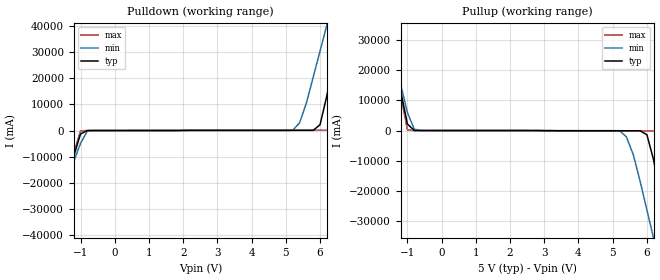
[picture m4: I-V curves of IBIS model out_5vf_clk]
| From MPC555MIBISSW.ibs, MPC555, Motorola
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| OUTPUT_5vf_clk(Full Strength, 90pf load)
[Model]   out_5vf_clk
Model_type   Output
Polarity   Non-Inverting
|   typ   min   max
C_comp   5.1000e-13   4.5360e-13   5.8450e-13
| CAP models
| typical : model= typ
| maximum : model= wcs
| minimum : model= bcs
[Voltage range]   5.0v   4.5v   5.5v
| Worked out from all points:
|   slope of the pulldown table from 0 to 0.75 V, typ, clamps not added: 187 ohm
|   slope of the pullup table from 0 to 0.75 V, typ, clamps not added: 744 ohm
|  typical: model = typ,  temp = 25,  vdd = 3.3, vddh = 5.0
|  maximum: model = bcs,  temp = -40, vdd = 3.6, vddh = 5.5
|  minimum: model = wcs,  temp = 150, vdd = 3.0, vddh = 4.5
[Pulldown]
|  Voltage   I(typ)   I(min)   I(max)
-5V       -319.1A    -223.2A    -410.6A
-1.8V     -50.29A    -40.81A    -60.01A
-1.6V     -36.77A    -31.17A    -42.83A
-1V       -1.324A    -4.896A    -109.6mA
5.2V      64.08mA    77.3mA     107mA
5.6V      64.46mA    10.49A     107.6mA
6V        2.23A      30.51A     108.4mA
6.2V      13.38A     40.53A     109mA
6.4V      27.52A     50.54A     113.6mA
6.6V      41.67A     60.57A     4.508A
7V        70.64A     85.73A     39.22A
10V       376.7A     302.1A     417A
[Pullup]
-5V       376.6A     266A       482A
-1.6V     41.61A     35.49A     48.13A
-1.4V     27.46A     25.48A     30.08A
-1V       2.165A     5.972A     209.1mA
-600mV    981.2uA    5.173mA    1.431mA
5.2V      -75.78mA   -60.19mA   -123.2mA
5.6V      -76.73mA   -7.957A    -124.7mA
6V        -1.399A    -26.39A    -126mA
6.4V      -23.34A    -45.68A    -130.1mA
6.6V      -36.85A    -55.33A    -3.582A
7V        -63.9A     -74.63A    -34.37A
10V       -319.2A    -255.2A    -353.5A
| RAMP models
| typical dv/dt : model=typ, temp=25
| maximum dv/dt : model=bcs, temp=-40
| minimum dv/dt : model=wcs, temp=150
|   typ   min   max
[Ramp]
dV/dt_r  1.78822/6.7468e-10   1.12787/1.59839e-09   2.39042/3.45165e-10
dV/dt_f  1.32072/2.3018e-10   0.787065/1.0136e-09   1.8222/2.45962e-10
